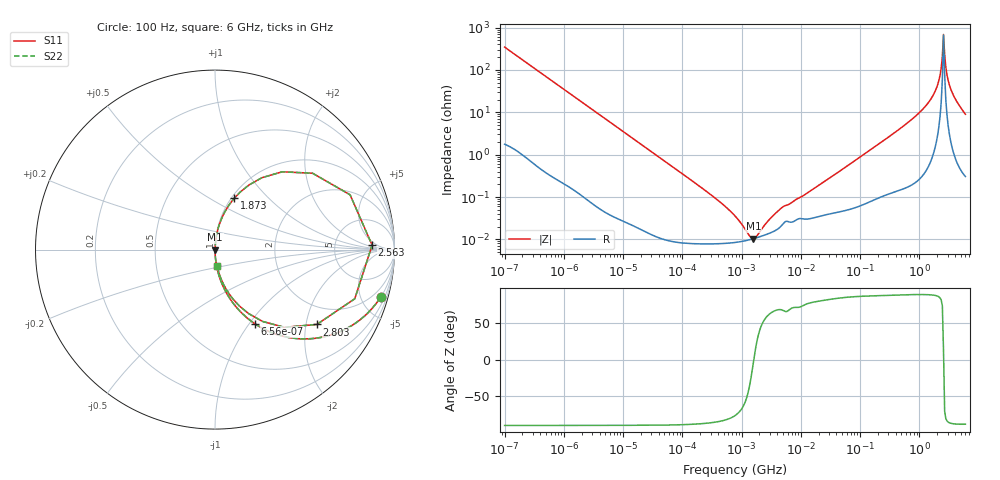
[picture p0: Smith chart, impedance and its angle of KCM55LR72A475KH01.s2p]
!Murata Part Number: KCM55LR72A475KH01
!These Parameters are Measured in Series Mode Connection
!Data Generated on Mar 13, 2026
!  o--ll--o
!Port1  Port2
!  o------o
!Operation Temp=25[degC], DC Bias Voltage=0[V]
!Freq. Start=100[Hz] Stop=6[GHz] 401[Steps]
# Hz S RI R 50
!Freq.(Hz) S11(Real) S11(Imag) S21(Real) S21(Imag) S12(Real) S12(Imag) S22(Real) S22(Imag)
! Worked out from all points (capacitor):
!   401 points, 100 Hz to 6 GHz, reference 50 ohm
!   read as one part in series: C = 4.57 uF near 109 Hz
!   lowest |Z| = 10.4 mohm at 1.586 MHz (marker M1)
!   series resonance near 1.609 MHz, so ESL is about 2.1 nH
!   S11 on the Smith chart (normalised r, x): 100 Hz: 1.04, -6.95; 656 Hz: 1.01, -1.07; 1.873 GHz: 1.03, +0.65; 2.563 GHz: 14, +3; 2.803 GHz: 1.40, -2.31; 6 GHz: 1.01, -0.18
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100  0.9224 -0.265  0.0776 0.265  0.0776 0.265  0.9224 -0.265
164  0.8178 -0.3831  0.1822 0.3831  0.1822 0.3831  0.8178 -0.3831
306  0.5649 -0.4931  0.4351 0.4931  0.4351 0.4931  0.5649 -0.4931
656  0.2231 -0.4136  0.7769 0.4136  0.7769 0.4136  0.2231 -0.4136
2008  0.0307 -0.1695  0.9693 0.1695  0.9693 0.1695  0.0307 -0.1695
40335  0.000186 -0.0088  0.9998 0.0088  0.9998 0.0088  0.000186 -0.0088
330837  7.94e-05 -0.00103  0.9999 0.00103  0.9999 0.00103  7.94e-05 -0.00103
774597  8.46e-05 -0.000348  0.9999 0.000348  0.9999 0.000348  8.46e-05 -0.000348
1585629  0.000104 -6.1e-06  0.9999 6.1e-06  0.9999 6.1e-06  0.000104 -6.1e-06
4643984  0.000205 0.000503  0.9998 -0.000503  0.9998 -0.000503  0.000205 0.000503
1.555665e7  0.000318 0.00146  0.9997 -0.00146  0.9997 -0.00146  0.000318 0.00146
3.124326e8  0.00191 0.0268  0.9981 -0.0268  0.9981 -0.0268  0.00191 0.0268
1.046602e9  0.0135 0.1026  0.9865 -0.1026  0.9865 -0.1026  0.0135 0.1026
1.873145e9  0.1077 0.2866  0.8923 -0.2866  0.8923 -0.2866  0.1077 0.2866
2.048624e9  0.1882 0.3593  0.8118 -0.3593  0.8118 -0.3593  0.1882 0.3593
2.240541e9  0.3741 0.4334  0.6259 -0.4334  0.6259 -0.4334  0.3741 0.4334
2.34314e9  0.5436 0.4255  0.4564 -0.4255  0.4564 -0.4255  0.5436 0.4255
2.562649e9  0.8754 0.0245  0.1246 -0.0245  0.1246 -0.0245  0.8754 0.0245
2.802721e9  0.5675 -0.4169  0.4325 0.4169  0.4325 0.4169  0.5675 -0.4169
3.065283e9  0.2653 -0.4003  0.7347 0.4003  0.7347 0.4003  0.2653 -0.4003
3.505958e9  0.1034 -0.2793  0.8966 0.2793  0.8966 0.2793  0.1034 -0.2793
6e9  0.011 -0.0889  0.989 0.0889  0.989 0.0889  0.011 -0.0889
